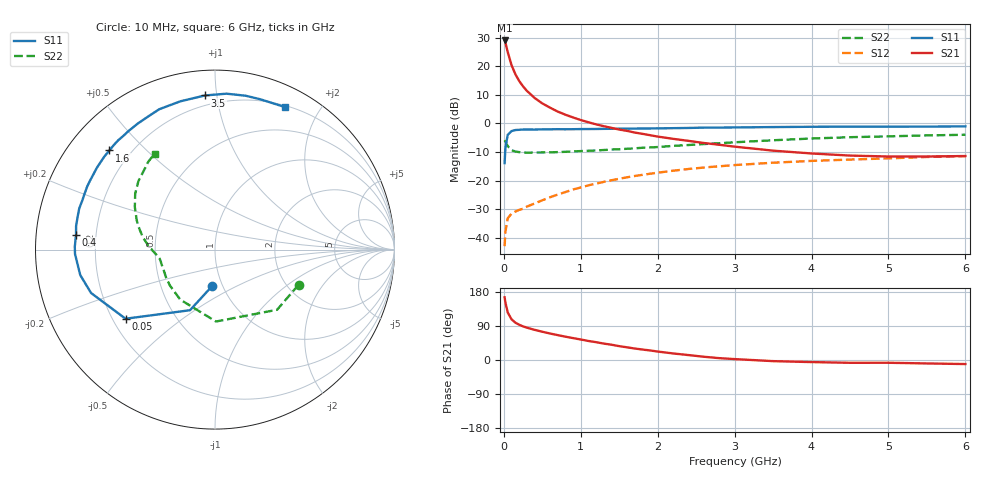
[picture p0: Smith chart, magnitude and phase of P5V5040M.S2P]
! SIEMENS Small Signal Semiconductors
! BFP183
! Si NPN RF Bipolar Junction Transistor in SOT143
! VCE = 0.5 V  IC = 40 mA
! Common Emitter S-Parameters:  March  1996
# GHz  S  MA  R  50
!  f  S11  S21  S12  S22
! GHz  MAG  ANG  MAG  ANG  MAG  ANG  MAG  ANG
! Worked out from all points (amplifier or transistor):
!   36 points, 10 MHz to 6 GHz, reference 50 ohm
!   highest |S21| = 29.0 dB at 10 MHz (marker M1)
!   |S21| within 3 dB of that: start of sweep to 40.94 MHz
!   unconditionally stable (mu >= 1): start of sweep to 20.91 MHz; 156.5 MHz to end of sweep
!   at 250 MHz: K = 1.35, MAG = 17.8 dB, |S12| = -29.8 dB
!   at 1.4 GHz: K = 2.07, MAG = 3.3 dB, |S12| = -19.9 dB
!   at 6 GHz: K = 1.48, MAG = -4.1 dB, |S12| = -11.5 dB
!   S11 on the Smith chart (normalised r, x): 10 MHz: 0.90, -0.38; 50 MHz: 0.25, -0.32; 400 MHz: 0.12, +0.05; 1.6 GHz: 0.12, +0.39; 3.5 GHz: 0.14, +0.93; 6 GHz: 0.22, +1.59
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0.01  0.2016 -94.0  28.19 165.3  0.0071 64.9  0.5052 -22.9
0.02  0.3652 -112.4  25.95 152.2  0.0125 60.4  0.4816 -44.1
0.05  0.6298 -142.3  17.82 125.8  0.0218 43.0  0.4007 -89.2
0.1  0.7316 -160.7  10.45 107.3  0.0263 33.2  0.3394 -124.8
0.15  0.764 -169.3  7.233 98.5  0.0286 32.8  0.3212 -141.4
0.2  0.7708 -174.3  5.493 93.0  0.0306 35.3  0.3138 -150.4
0.25  0.7803 -178.2  4.432 88.7  0.0322 37.3  0.309 -155.7
0.3  0.7813 178.8  3.699 85.3  0.035 40.7  0.3078 -159.6
0.4  0.7786 174.0  2.781 79.6  0.0396 45.3  0.3087 -164.4
0.5  0.7849 170.4  2.232 74.6  0.0451 47.9  0.3093 -167.4
0.6  0.7869 166.6  1.883 69.9  0.0509 50.6  0.311 -169.6
0.7  0.7905 163.1  1.608 65.7  0.0567 52.3  0.314 -171.2
0.9  0.7901 157.2  1.268 57.8  0.0696 53.6  0.3232 -173.5
1.1  0.7953 151.1  1.044 50.2  0.0824 53.2  0.3312 -175.8
1.3  0.8007 145.3  0.891 43.3  0.0947 52.2  0.3414 -177.9
1.6  0.807 136.8  0.739 33.5  0.1137 49.9  0.359 178.9
2.2  0.8236 121.5  0.536 17.3  0.1483 42.9  0.4033 171.0
2.8  0.8427 107.4  0.422 4.9  0.1774 35.0  0.4494 162.5
3.5  0.8606 93.7  0.333 -3.0  0.2048 26.2  0.5059 152.0
4.5  0.8741 78.8  0.273 -7.4  0.2324 14.6  0.5724 138.2
5.5  0.877 68.3  0.263 -9.1  0.2581 4.9  0.6148 127.2
6  0.8849 63.7  0.268 -10.7  0.2667 -0.2  0.6315 122.2
